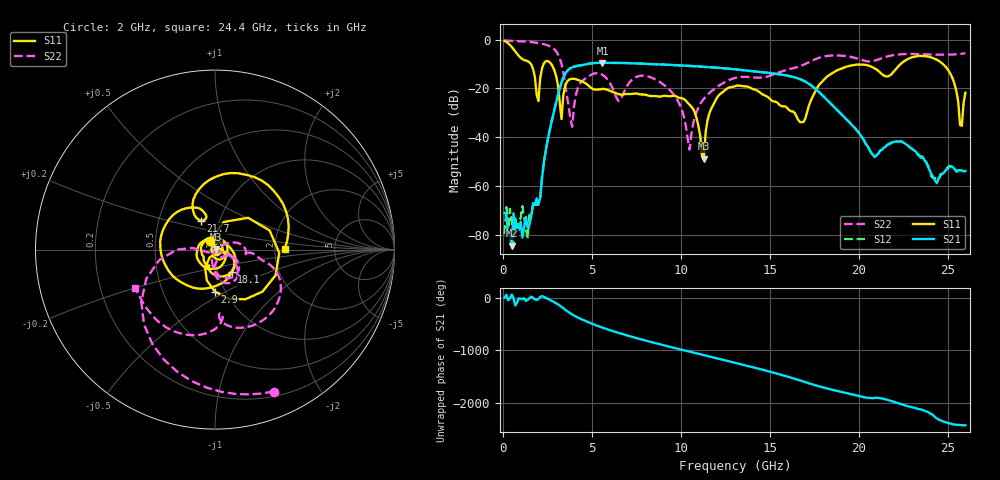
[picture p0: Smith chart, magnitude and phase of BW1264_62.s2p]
!Keysight Technologies,N5245B,MY57181159,A.13.60.06
!Date: Friday, December 18, 2020 23:55:17
!Correction: S11(Full 2 Port(1,2))
!S21(Full 2 Port(1,2))
!S12(Full 2 Port(1,2))
!S22(Full 2 Port(1,2))
!S2P File: Measurements: S11, S21, S12, S22:
# Hz S  dB  R 50
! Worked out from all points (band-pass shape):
!   260 points, 100 MHz to 26 GHz, reference 50 ohm
!   highest |S21| = -9.49 dB at 5.6 GHz (marker M1); lowest = -84.6 dB at 500 MHz (marker M2)
!   |S21| within 3 dB of the highest: 3.663 GHz to 13.45 GHz (9.789 GHz wide, 114 % of centre)
!   lowest |S11| = -48.8 dB at 11.3 GHz (marker M3), VSWR 1.01, Z = 50.4 + j0.0722 ohm
!   |S11| at or under -10 dB: 1.574 GHz to 2.292 GHz (717.3 MHz wide, 37.1 % of centre); 2.719 GHz to 22.36 GHz (19.64 GHz wide, 157 % of centre); 24.73 GHz to end of sweep
!   |S22| runs from -45.1 to -0.3 dB; largest |S21 - S12| = 0.00059
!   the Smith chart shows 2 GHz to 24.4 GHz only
!   S11 on the Smith chart (normalised r, x): 2 GHz: 0.94, +0.09; 2.9 GHz: 0.90, -0.44; 18.1 GHz: 1.16, -0.30; 21.7 GHz: 0.82, +0.27; 24.4 GHz: 2.26, +0.02
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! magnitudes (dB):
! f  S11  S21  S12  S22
! 100 MHz  -0.5  -71.1  -79.8  -0.3
! 500 MHz  -3.0  -84.6  -74.8  -0.5
! 2 GHz  -25.2  -67.7  -67.6  -1.4
! 2.3 GHz  -9.8  -50.9  -50.9  -1.8
! 2.9 GHz  -12.6  -28.6  -28.6  -4.0
! 3.3 GHz  -32.6  -17.5  -17.5  -10.0
! 3.9 GHz  -16.1  -11.3  -11.3  -35.7
! 4.5 GHz  -17.3  -10.4  -10.4  -16.7
! 5.6 GHz  -20.2  -9.5  -9.5  -14.4
! 8.8 GHz  -23.4  -10.1  -10.1  -17.3
! 10.5 GHz  -26.7  -10.8  -10.8  -45.1
! 11.3 GHz  -48.8  -11.1  -11.1  -24.3
! 11.7 GHz  -28.5  -11.3  -11.3  -21.3
! 13.1 GHz  -18.9  -12.2  -12.2  -15.6
! 16.7 GHz  -33.8  -16.2  -16.2  -10.9
! 17.4 GHz  -23.6  -19.2  -19.1  -8.5
! 18.1 GHz  -16.1  -23.8  -23.8  -6.8
! 21.7 GHz  -14.9  -42.9  -42.7  -6.7
! 24.4 GHz  -8.2  -58.9  -57.4  -6.1
! 25.3 GHz  -16.3  -52.4  -52.0  -6.1
! 25.7 GHz  -35.0  -53.6  -53.5  -5.8
! 26 GHz  -21.8  -53.9  -54.1  -5.6
